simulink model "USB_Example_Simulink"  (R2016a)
settings: Solver=VariableStepAuto  StartTime=0.0  StopTime=10.0  RelTol=1e-3
libraries: sldrtlib x1

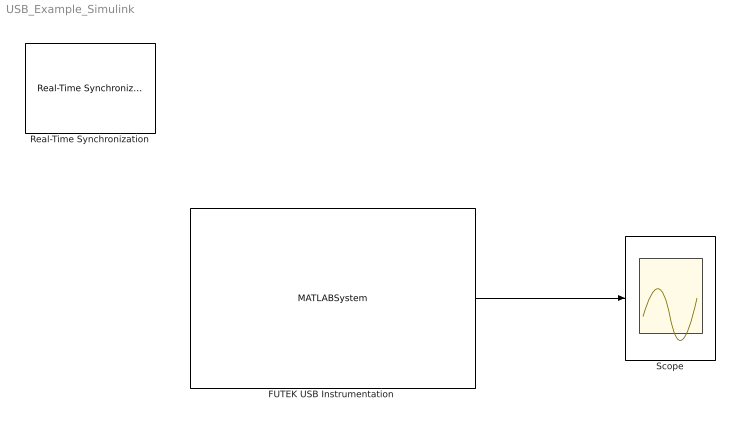
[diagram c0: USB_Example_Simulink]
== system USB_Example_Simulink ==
  "FUTEK USB Instrumentation " : MATLABSystem  System=USB_Sensor_Simulink_Object  SerialNumber=591916  SimulateUsing=Interpreted execution
  Real-Time Synchronization : sldrtlib/Real-Time Synchronization  SampleTime=0.1  MaxMissedTicks=10  ShowMissedTicks=off  YieldWhenWaiting=off
  Scope : Scope
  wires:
  "FUTEK USB Instrumentation "/1 -> Scope/1
